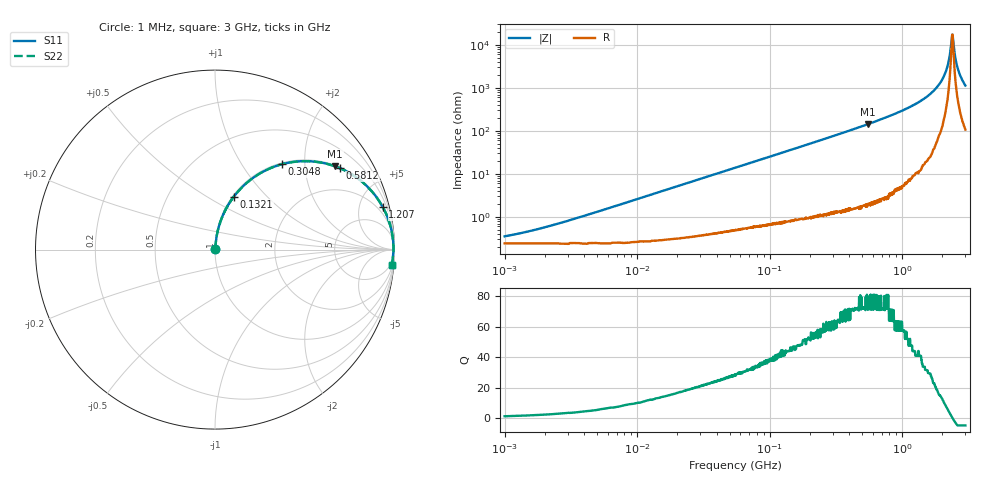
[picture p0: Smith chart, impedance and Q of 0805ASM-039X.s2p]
!s-Parameter Generated by FASTRON Sdn. Bhd.
!FASTRON P/N : 0805ASM-039X
!Keysight Technologies: E4991B_MY54100416_A.01.15
!Date: Fri Jun 19 14:48:56 2026
!Version  :Rev00  Fri Jun 19 14:48:56 2026
!Data & Calibration Information:
!Freq  S11  S21  S12  S22
!PortZ  Port1:50+j0  Port2:50+j0
!When reading reference impedance value at option line is always used.
! Remarks : This data is being provided solely for informational purposes.
# Hz S dB R 50
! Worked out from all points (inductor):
!   1601 points, 1 MHz to 3 GHz, reference 50 ohm
!   read as one part in series: L = 41.1 nH near 2.762 MHz
!   highest Q = 72.4 at 550.1 MHz (marker M1), where L = 41.3 nH
!   self-resonance near 2.383 GHz
!   S11 on the Smith chart (normalised r, x): 1 MHz: 1.00, +0.01; 132.1 MHz: 1.01, +0.66; 304.8 MHz: 1.03, +1.53; 581.2 MHz: 1.04, +3.04; 1.207 GHz: 1.18, +7.85; 3 GHz: 3, -23
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1000000  -49.10 46.7  -0.02 -0.1  -0.02 -0.1  -49.10 46.7
3804036  -39.90 75.7  -0.02 -0.6  -0.02 -0.6  -39.90 75.7
1.447069e7  -28.60 83.5  -0.03 -2.1  -0.03 -2.1  -28.60 83.5
5.504702e7  -17.30 80.1  -0.12 -7.9  -0.12 -7.9  -17.30 80.1
1.321429e8  -10.10 70.5  -0.51 -18.2  -0.51 -18.2  -10.10 70.5
2.083556e8  -6.77 61.6  -1.11 -27.3  -1.11 -27.3  -6.77 61.6
3.047674e8  -4.38 51.9  -2.08 -37.1  -2.08 -37.1  -4.38 51.9
5.500551e8  -1.79 34.7  -4.89 -54.5  -4.89 -54.5  -1.79 34.7
5.81181e8  -1.62 33.1  -5.25 -56.1  -5.25 -56.1  -1.62 33.1
7.925923e8  -0.87 24.5  -7.65 -64.7  -7.65 -64.7  -0.87 24.5
1.206698e9  -0.32 14.2  -12.20 -74.5  -12.20 -74.5  -0.32 14.2
1.581072e9  -0.14 8.5  -16.60 -79.6  -16.60 -79.6  -0.14 8.5
1.950859e9  -0.07 4.2  -22.70 -81.8  -22.70 -81.8  -0.07 4.2
2.167021e9  -0.05 2.0  -28.80 -79.7  -28.80 -79.7  -0.05 2.0
2.23307e9  -0.05 1.4  -31.80 -76.6  -31.80 -76.6  -0.05 1.4
2.324278e9  -0.05 0.6  -38.50 -61.8  -38.50 -61.8  -0.05 0.6
2.383164e9  -0.05 0.1  -44.60 -15.2  -44.60 -15.2  -0.05 0.1
2.455801e9  -0.05 -0.5  -39.10 57.6  -39.10 57.6  -0.05 -0.5
2.568929e9  -0.06 -1.5  -31.40 74.9  -31.40 74.9  -0.06 -1.5
2.673854e9  -0.07 -2.4  -27.60 78.3  -27.60 78.3  -0.07 -2.4
2.839331e9  -0.08 -3.7  -23.80 79.7  -23.80 79.7  -0.08 -3.7
3e9  -0.10 -5.0  -21.20 79.6  -21.20 79.6  -0.10 -5.0
